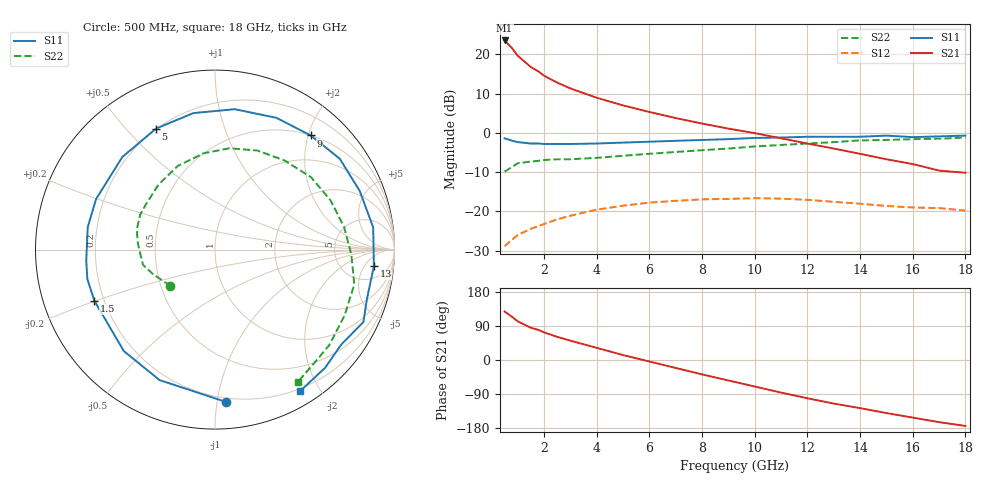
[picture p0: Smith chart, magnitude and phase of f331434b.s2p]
!ATF-33143
!S-PARAMETERS at Vds=4V  Id=80mA.  LAST UPDATED 09-29-99
# ghz s ma r 50
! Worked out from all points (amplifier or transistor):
!   23 points, 500 MHz to 18 GHz, reference 50 ohm
!   highest |S21| = 23.5 dB at 500 MHz (marker M1)
!   |S21| within 3 dB of that: start of sweep to 899.4 MHz
!   unconditionally stable (mu >= 1): 3.519 GHz to end of sweep
!   at 1.5 GHz: K = 0.73, MSG = 20.6 dB, |S12| = -24.4 dB
!   at 7 GHz: K = 1.11, MAG = 8.5 dB, |S12| = -17.3 dB
!   at 18 GHz: K = 1.35, MAG = 1.3 dB, |S12| = -19.8 dB
!   lowest NFmin = 0.11 dB at 500 MHz
!   S11 on the Smith chart (normalised r, x): 500 MHz: 0.17, -1.06; 1.5 GHz: 0.16, -0.20; 5 GHz: 0.20, +0.61; 9 GHz: 0.50, +2.04; 13 GHz: 10, -9; 18 GHz: 0.17, -1.75
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0.5  0.85 -86.0  14.98 128.0  0.036 52.0  0.32 -141.0
0.8  0.79 -113.0  11.75 113.0  0.044 45.0  0.37 -158.0
1  0.76 -132.0  9.56 102.0  0.05 40.0  0.41 -168.0
1.5  0.73 -157.0  6.86 85.0  0.06 36.0  0.43 176.0
1.8  0.73 -167.0  5.99 79.0  0.065 34.0  0.44 170.0
2  0.72 -175.0  5.32 73.0  0.069 32.0  0.45 165.0
2.5  0.72 170.0  4.35 61.0  0.079 29.0  0.46 155.0
3  0.72 157.0  3.67 51.0  0.088 24.0  0.46 147.0
4  0.73 135.0  2.79 32.0  0.105 14.0  0.48 131.0
5  0.75 116.0  2.23 13.0  0.118 3.0  0.51 114.0
6  0.77 99.0  1.84 -4.0  0.129 -9.0  0.54 97.0
7  0.79 82.0  1.54 -21.0  0.136 -22.0  0.57 82.0
8  0.81 65.0  1.31 -38.0  0.142 -34.0  0.6 67.0
9  0.83 50.0  1.13 -54.0  0.144 -47.0  0.63 52.0
10  0.86 36.0  0.99 -70.0  0.147 -60.0  0.67 37.0
11  0.87 22.0  0.85 -86.0  0.145 -73.0  0.7 23.0
12  0.89 8.0  0.73 -101.0  0.14 -85.0  0.73 10.0
13  0.89 -6.0  0.63 -115.0  0.132 -97.0  0.76 -2.0
14  0.89 -18.0  0.54 -127.0  0.125 -106.0  0.8 -14.0
15  0.92 -26.0  0.46 -140.0  0.117 -116.0  0.81 -27.0
16  0.88 -37.0  0.4 -152.0  0.112 -126.0  0.83 -40.0
18  0.92 -59.0  0.31 -174.0  0.102 -144.0  0.87 -58.0
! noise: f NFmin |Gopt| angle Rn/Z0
0.5  0.11  0.7  41  0.07
0.9  0.16  0.64  61  0.06
1.5  0.25  0.55  91  0.06
1.8  0.3  0.51  106  0.05
2.5  0.41  0.42  139  0.03
3  0.49  0.39  160  0.03
5  0.8  0.43  -134  0.08
6  0.96  0.5  -110  0.15
8  1.27  0.66  -72  0.47
10  1.59  0.65  -39  0.98
